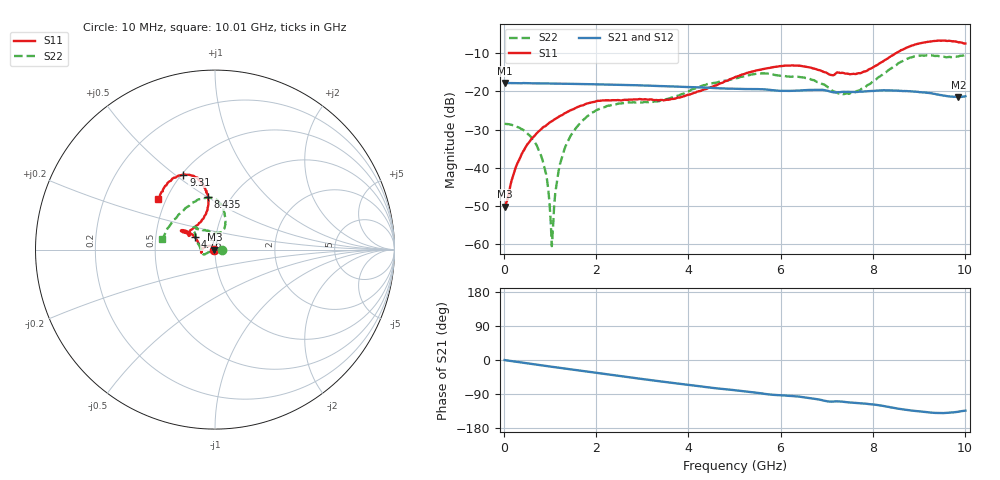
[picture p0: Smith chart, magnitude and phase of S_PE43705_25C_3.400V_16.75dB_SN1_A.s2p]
! Device ID: PE43705
! Serial: 1
! Insertion: A
! Impedance: 50 ohm
! Temp: 25C
! VDD: 3.400V
! Attenuation Step: 16.75dB
#  Hz  S  RI  R  50
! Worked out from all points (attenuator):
!   401 points, 10 MHz to 10.01 GHz, reference 50 ohm
!   highest |S21| = -17.82 dB at 10 MHz (marker M1); lowest = -21.5 dB at 9.86 GHz (marker M2)
!   lowest |S11| = -50.1 dB at 10 MHz (marker M3), VSWR 1.01, Z = 49.7 + j0.033 ohm
!   |S11| at or under -10 dB: start of sweep to 8.512 GHz
!   |S22| runs from -60.5 to -10.4 dB; largest |S21 - S12| = 0.0015
!   S11 on the Smith chart (normalised r, x): 10 MHz: 0.99, +0.00; 4.76 GHz: 0.79, +0.11; 8.435 GHz: 0.78, +0.50; 9.31 GHz: 0.51, +0.54; 10.01 GHz: 0.45, +0.31
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1e7  -0.0031 0.000332  0.1285 -0.000516  0.1286 -0.000487  0.0376 3.3e-05
3.1e8  -0.00536 0.0109  0.1271 -0.0121  0.1272 -0.0121  0.0335 0.0038
7.35e8  -0.0203 0.0213  0.1238 -0.028  0.1239 -0.0279  0.0169 0.0057
9.1e8  -0.0284 0.0215  0.1219 -0.0344  0.1219 -0.0343  0.00768 0.00318
1.01e9  -0.0337 0.0213  0.1205 -0.0379  0.1205 -0.0378  0.0016 0.00121
1.035e9  -0.0347 0.021  0.1201 -0.0388  0.1202 -0.0387  0.000189 0.000929
1.085e9  -0.0374 0.0204  0.1194 -0.0403  0.1193 -0.0403  -0.00314 -0.000295
1.16e9  -0.0409 0.0198  0.1184 -0.0428  0.1184 -0.0428  -0.00731 -0.0018
1.26e9  -0.0454 0.0181  0.1169 -0.0462  0.1169 -0.0462  -0.0134 -0.00413
1.685e9  -0.0646 0.00766  0.1091 -0.0596  0.1091 -0.0597  -0.0376 -0.0155
2.26e9  -0.0757 -0.0105  0.0961 -0.0757  0.0962 -0.0756  -0.0586 -0.0278
3.36e9  -0.0761 -0.00721  0.0656 -0.0971  0.0658 -0.097  -0.0742 -0.00384
4.76e9  -0.1118 0.0697  0.0252 -0.106  0.0254 -0.106  -0.1095 0.0815
5.01e9  -0.1277 0.0847  0.0187 -0.1061  0.019 -0.1062  -0.1136 0.094
5.985e9  -0.1834 0.1087  -0.00519 -0.1012  -0.00478 -0.1012  -0.1039 0.1212
6.685e9  -0.1762 0.0958  -0.0209 -0.1022  -0.0207 -0.1021  -0.0852 0.1122
7.435e9  -0.122 0.1184  -0.0359 -0.0917  -0.0354 -0.0916  0.00912 0.0939
8.36e9  -0.0366 0.2766  -0.0576 -0.0851  -0.0579 -0.0857  0.0561 0.1848
8.435e9  -0.0389 0.2939  -0.06 -0.083  -0.0602 -0.0837  0.0537 0.1999
9.31e9  -0.176 0.4178  -0.0704 -0.0605  -0.0702 -0.0605  -0.1012 0.2749
9.86e9  -0.2905 0.3253  -0.0611 -0.0578  -0.0611 -0.0575  -0.2552 0.1285
1.001e10  -0.3149 0.28  -0.0595 -0.0623  -0.06 -0.0621  -0.2942 0.0615
